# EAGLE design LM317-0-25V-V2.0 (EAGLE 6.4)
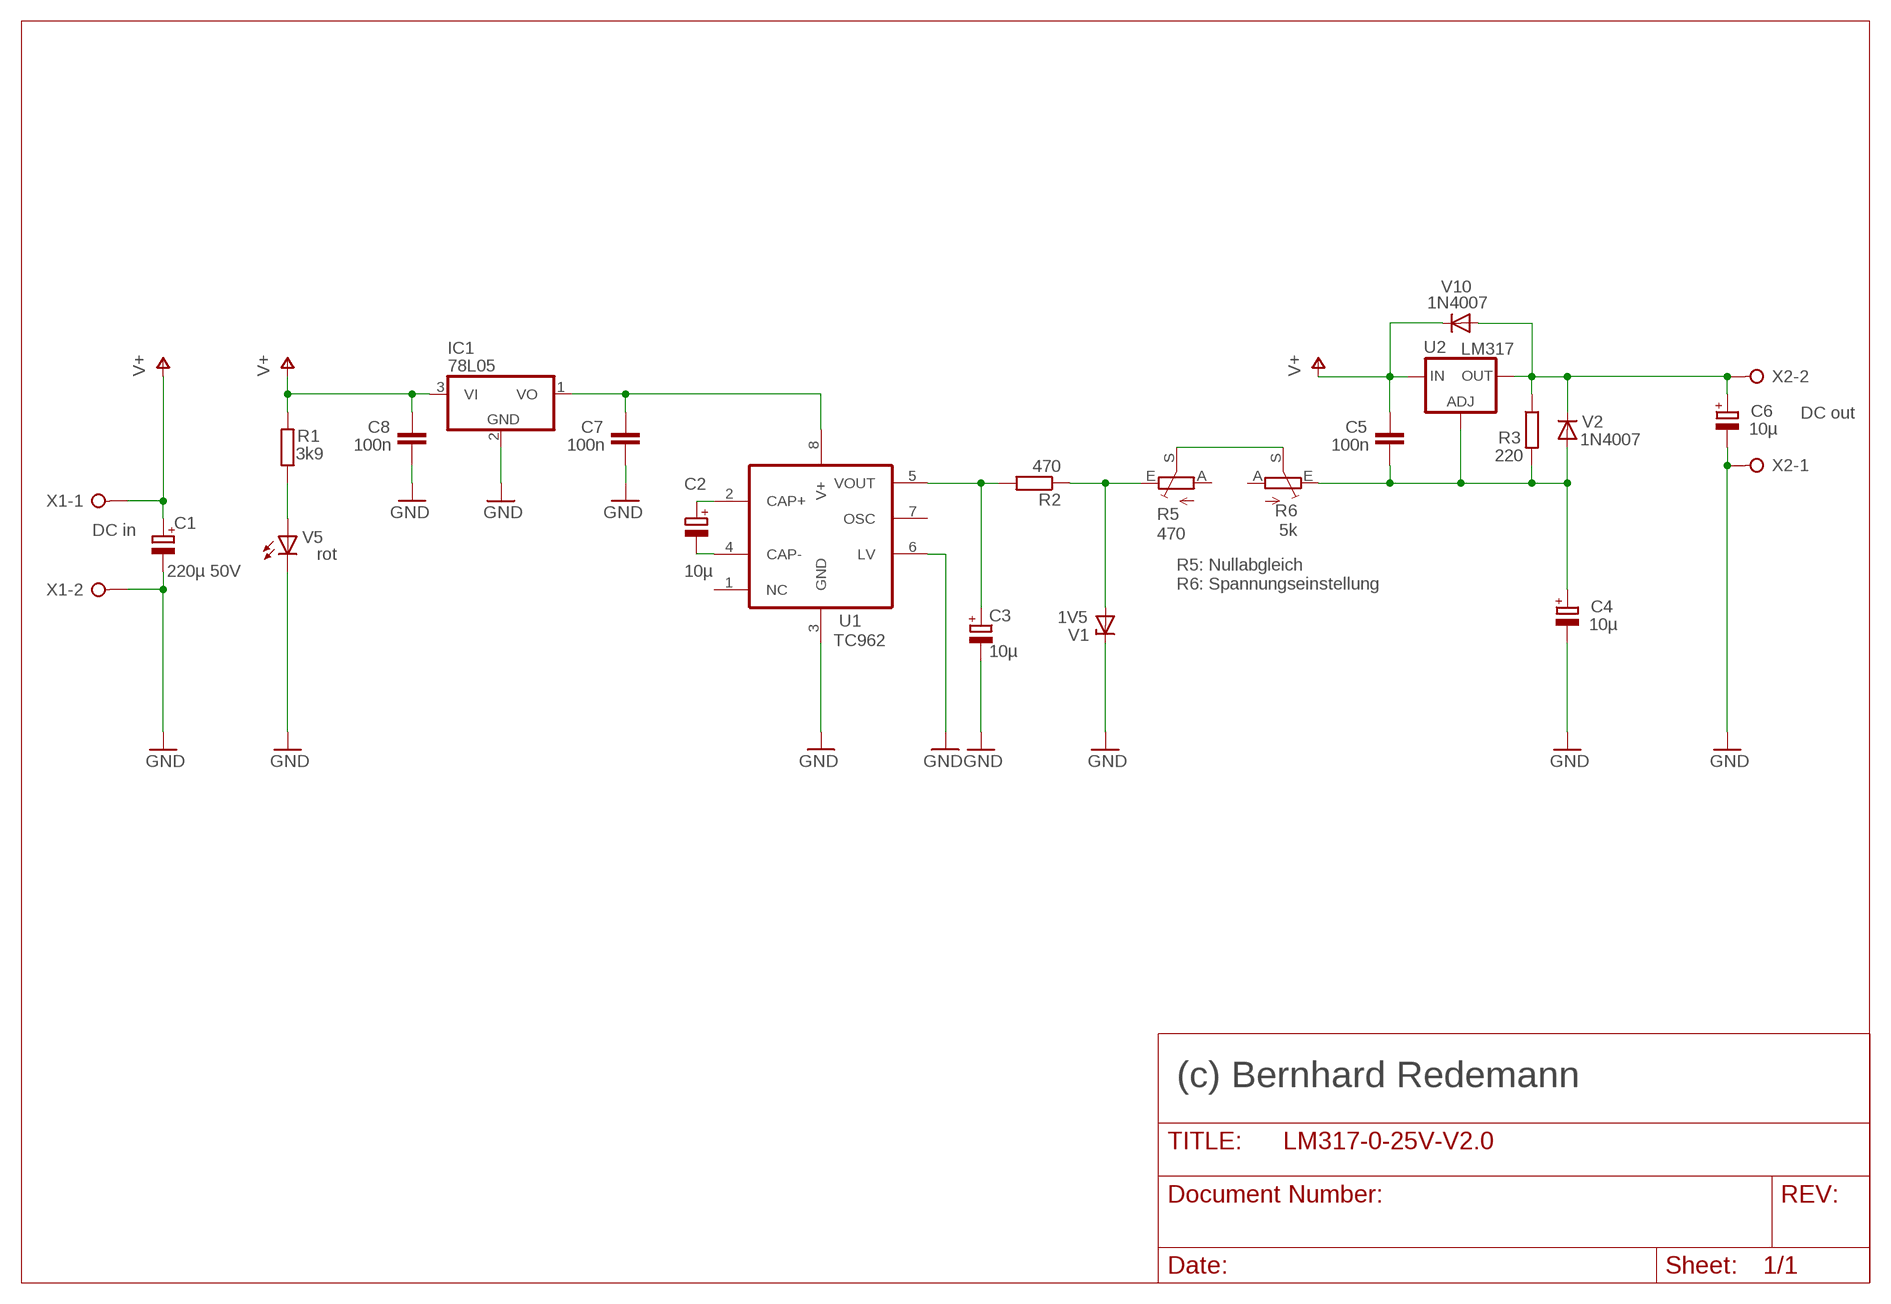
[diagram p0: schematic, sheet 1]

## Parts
C1  220µ 50V  CPOL-EUE5-10.5  [E5-10,5]
C2  10µ  CPOL-EUE1.8-4  [E1,8-4]
C3  10µ  CPOL-EUE1.8-4  [E1,8-4]
C4  10µ  CPOL-EUE1.8-4  [E1,8-4]
C5  100n  C-EU025-024X044  [C025-024X044]
C6  10µ  CPOL-EUE1.8-4  [E1,8-4]
C7  100n  C-EU025-024X044  [C025-024X044]
C8  100n  C-EU025-024X044  [C025-024X044]
IC1  78L05  78L05Z  [TO92]
R1  3k9  R-EU_0309/10  [0309/10]
R2  470  R-EU_0204/7  [0204/7]
R3  220  R-EU_0204/7  [0204/7]
R5  470  TRIM_EU-B64Y  [B64Y]
R6  5k  TRIM_EU-B64Y  [B64Y]
U1  TC962  ICL7660CPA  [DIL08]
U2  LM317  LM317TS  [317TS]
V1  1V5  ZPD  [DO35Z10]
V2  1N4007  1N4004  [DO41-10]
V5  rot  LED3MM  [LED3MM]
V10  1N4007  1N4004  [DO41-10]
X1  DC in  W237-02P  [W237-132]
X2  DC out  W237-02P  [W237-132]

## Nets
GND: C1.- C3.- C4.- C6.- C7.2 C8.2 IC1.2(GND) U1.3(GND) U1.6(LV) V1.C V5.K(C) X1.2 X2.1
N$1: C7.1 IC1.1(VO) U1.8(V+)
N$4: C6.+ R3.1 U2.2(OUT) V2.C V10.A X2.2
N$6: C2.+ U1.2(CAP+)
N$7: C2.- U1.4(CAP-)
N$8: R1.1 V5.A
N$9: C3.+ R2.2 U1.5(VOUT)
N$11: R2.1 R5.E V1.A
N$12: C4.+ C5.2 R3.2 R6.E U2.1(ADJ) V2.A
N$13: R5.S R6.S
V+: C1.+ C5.1 C8.1 IC1.3(VI) R1.2 U2.3(IN) V10.C X1.1
Unconnected: R5.A R6.A U1.1(NC) U1.7(OSC)

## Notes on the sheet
- R5: Nullabgleich
  R6: Spannungseinstellung
- (c) Bernhard Redemann

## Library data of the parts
C1-C4 C6 = resistor:CPOL-EU: POLARIZED CAPACITOR, European symbol
C5 C7 C8 = resistor:C-EU: CAPACITOR, European symbol
IC1 = linear:78*: Positive VOLTAGE REGULATOR Source: http://cache.national.com/ds/LM/LM78L05.pdf http://www.fairchildsemi.com/ds/LM/LM7805.pdf
R1-R3 = rcl:R-EU_: RESISTOR, European symbol
R5 R6 = pot:TRIM_EU-: POTENTIOMETER
U1 = maxim:ICL7660CPA: VOLTAGE CONVERTER; MF: INTERSIL; MPN: ICL7660CPA; OC_FARNELL: 1018170; OC_NEWARK: 06F7441
U2 = v-reg:LM317TS: VOLTAGE REGULATOR
V1 = diode:ZPD: Z DIODE
V2 V10 = diode:1N4004: DIODE
V5 = 01-Parts1:LED: LED
X1 X2 = con-wago-508:W237-02P: WAGO SREW CLAMP; OC_FARNELL: unknown; OC_NEWARK: unknown

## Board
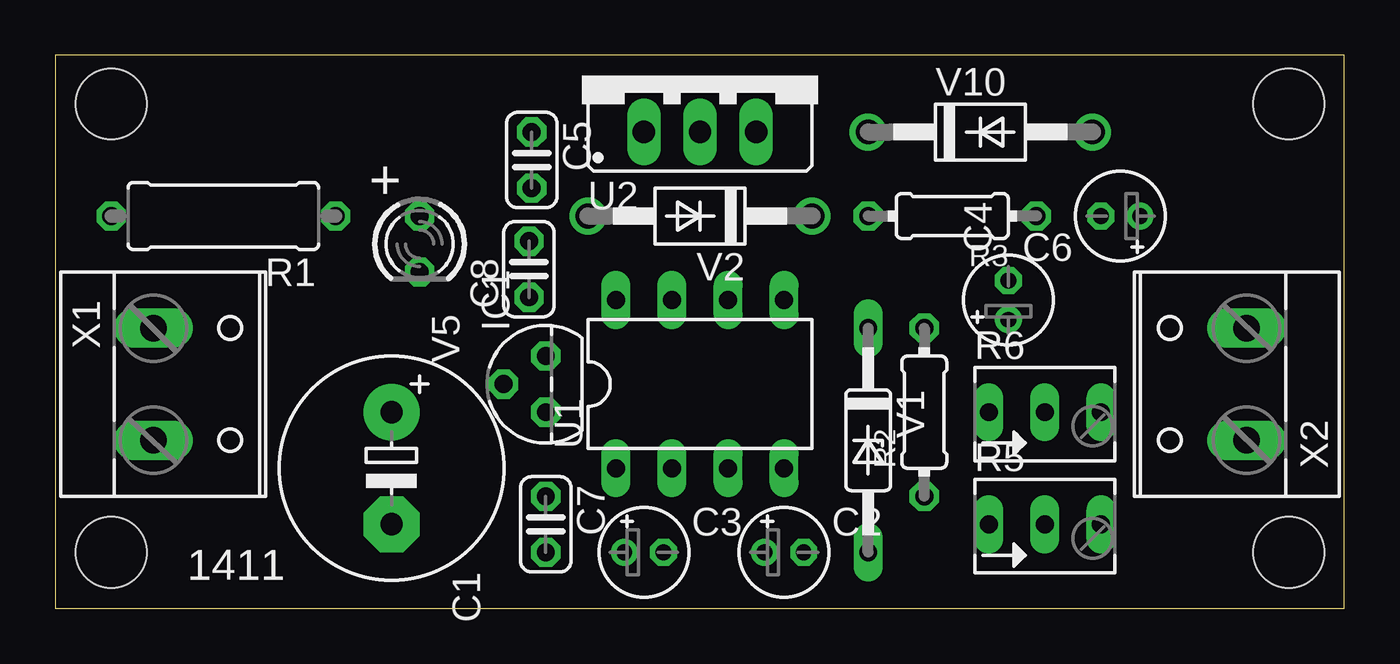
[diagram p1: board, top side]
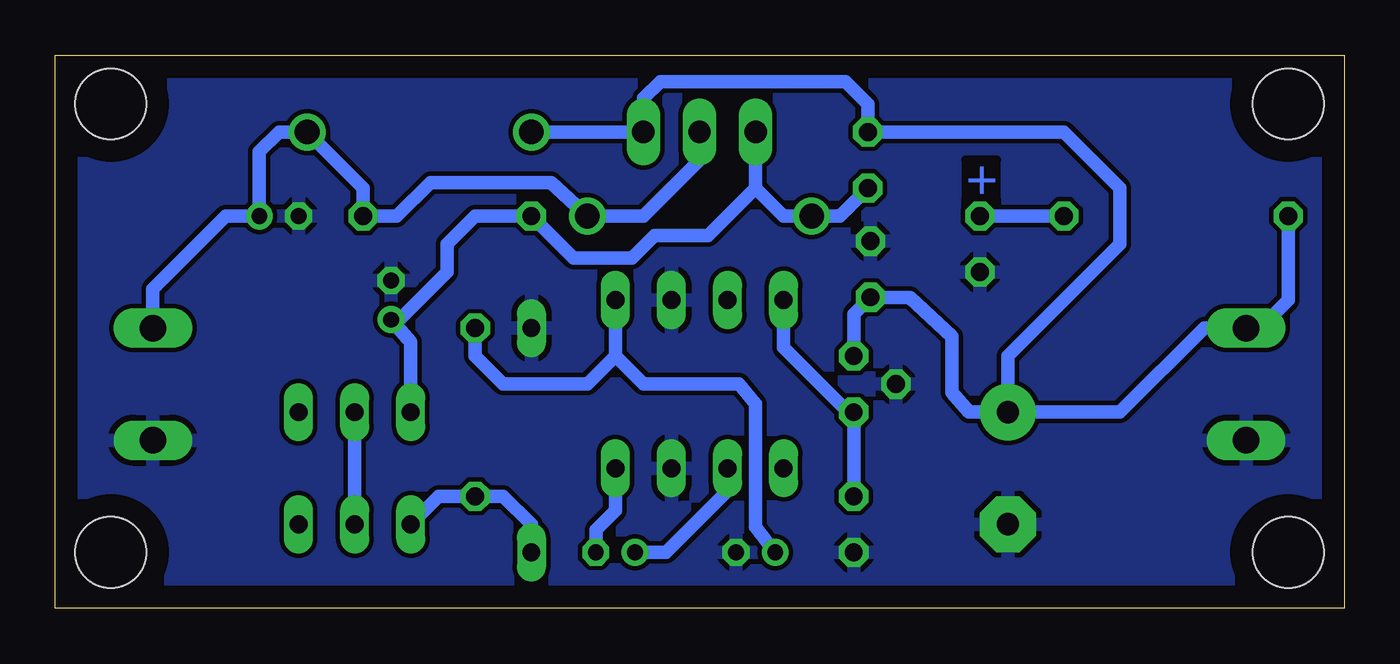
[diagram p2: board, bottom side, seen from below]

Size 58.4 x 25.07 mm. Coordinates in mm from the lower left corner, seen from the top.
Outline: 0,0 58.4,0 58.4,25.07 0,25.07 0,0
Copper layers (1*16): Top 0.035mm / dielectric 1.5mm / Bottom 0.035mm
Design rules "default": minimum track width 10mil, minimum drill 24mil, track to track 8mil, track to pad 8mil, pad to pad 8mil, via to via 8mil, smd to smd 8mil, copper to edge 40mil, drill to drill 8mil, minimum pad ring 10mil, minimum via ring 8mil, stop-mask expansion 4mil, vias tented up to drill 0mil, thermal gap 10mil
Holes 3.2 mm at 2.54,2.54 55.88,2.54 2.54,22.86 55.88,22.86

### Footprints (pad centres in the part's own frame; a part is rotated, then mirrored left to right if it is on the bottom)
E5-10,5 = drill 1.016 pad 2.54: + -2.54,0 | drill 1.016 pad 2.54 octagon: - 2.54,0
E1,8-4 = drill 0.711 pad 1.168: + -0.889,0 | drill 0.711 pad 1.168 octagon: - 0.889,0
C025-024X044 = drill 0.813 octagon: 1 -1.27,0; 2 1.27,0
TO92 = drill 0.813 octagon: 1 -1.27,0; 2 0,1.905; 3 1.27,0
0309/10 = drill 0.813 octagon: 1 -5.08,0; 2 5.08,0
0204/7 = drill 0.813 octagon: 1 -3.81,0; 2 3.81,0
B64Y = drill 0.813 long: A 2.54,0; E -2.54,0; S 0,0
DIL08 = drill 0.813 long: 1 -3.81,-3.81; 2 -1.27,-3.81; 3 1.27,-3.81; 4 3.81,-3.81; 5 3.81,3.81; 6 1.27,3.81; 7 -1.27,3.81; 8 -3.81,3.81
317TS = drill 1.016 long: 1 -2.54,-2.54; 2 0,-2.54; 3 2.54,-2.54
DO35Z10 = drill 0.813 long: A 5.08,0; C -5.08,0
DO41-10 = drill 1.118: A 5.08,0; C -5.08,0
LED3MM = drill 0.813 octagon: A -1.27,0; K 1.27,0
W237-132 = drill 1.194 long: 1 -2.54,-0.635; 2 2.54,-0.635

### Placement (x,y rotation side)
C1  15.24,6.35 270 top
C2  33.02,2.54 0 top
C3  26.67,2.54 0 top
C4  43.18,13.97 90 top
C5  21.59,20.32 270 top
C6  48.26,17.78 180 top
C7  22.23,3.81 270 top
C8  21.46,15.37 90 top
IC1  22.23,10.16 90 top
R1  7.62,17.78 180 top
R2  39.37,8.89 90 top
R3  40.64,17.78 180 top
R5  44.83,3.81 0 top
R6  44.83,8.89 0 top
U1  29.21,10.16 0 top
U2  29.21,24.13 0 top
V1  36.83,7.62 270 top
V2  29.21,17.78 180 top
V5  16.51,16.51 270 top
V10  41.91,21.59 0 top
X1  5.08,10.16 270 top
X2  53.34,10.16 90 top

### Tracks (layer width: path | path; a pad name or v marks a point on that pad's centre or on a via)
GND
  pour Bottom: 0,24.64 0,0 58.17,0 58.17,24.64
N$1
  Bottom 0.61: C7.1 IC1.1 22.48,8.89 25.4,11.81 U1.8
N$4
  Bottom 0.61: X2.2 53.98,14.48 50.67,17.78 C6.+ 49.15,20.7 48.26,21.59 V10.A 44.45,19.05 R3.1 42.93,17.78 41.4,19.3 35.94,19.3 V2.C 31.75,17.78 29.21,20.32 U2.2
N$6
  Bottom 0.61: C2.+ 30.73,2.54 27.94,5.33 U1.2
N$7
  Bottom 0.61: C2.- 33.91,3.56 33.02,4.45 U1.4
N$8
  Bottom 0.61: R1.1 V5.A
N$9
  Bottom 0.61: C3.+ 26.67,3.68 26.67,9.27 27.43,10.16 31.75,10.16 33.02,11.43 | 33.02,11.43 U1.5 | R2.2 39.37,11.43 38.1,10.16 34.29,10.16 33.02,11.43
N$11
  Bottom 0.61: R5.E 41.02,5.08 R2.1 38.1,5.08 36.83,3.81 V1.A
N$12
  Bottom 0.61: U2.1 26.67,19.05 | 26.67,19.05 25.4,17.78 V2.A 22.86,17.78 C5.2 | 26.67,19.05 28.83,16.89 31.24,16.89 32.26,15.88 34.92,15.88 R3.2 39.37,17.78 40.64,16.51 40.64,15.24 42.8,13.08 C4.+ 42.29,12.06 R6.E
N$13
  Bottom 0.61: R5.S R6.S
V+
  Bottom 0.61: R1.2 2.54,13.97 3.81,12.7 X1.1 6.35,12.7 10.16,8.89 C1.+ | C1.+ 15.24,11.43 10.16,16.51 10.16,19.05 12.7,21.59 C5.1 21.59,22.86 22.61,23.88 30.99,23.88 31.75,23.11 U2.3 V10.C | IC1.3 22.23,13.34 C8.1 19.68,14.1 17.78,12.32 17.78,9.78 17.02,8.89 C1.+

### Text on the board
Bottom: +
tPlace: + | 1411
tValues: LNR317 V2.0 | b-redemann.de | + | +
